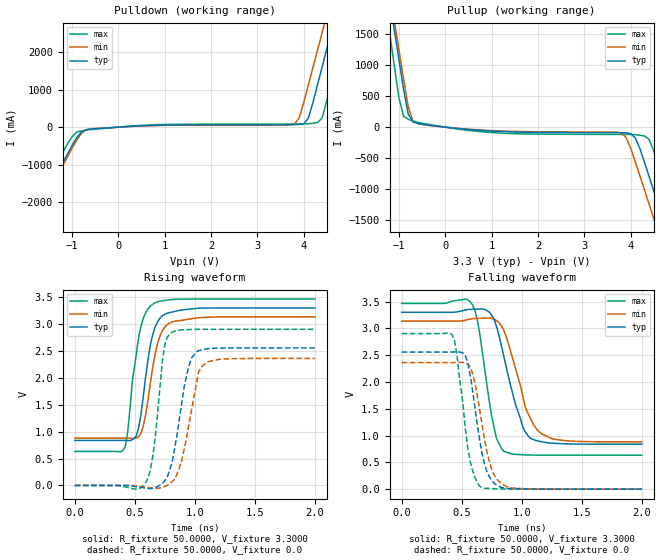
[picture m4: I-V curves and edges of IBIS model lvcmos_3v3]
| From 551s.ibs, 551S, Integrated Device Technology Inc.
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|   Model LVCMOS_3V3
[Model]  lvcmos_3v3
Model_type Output
Polarity   Non-Inverting
Vmeas =  1.6500V
Cref =   5.0000pF
Rref =   50.0000
Vref =   1.6500V
C_comp   2.0000pF   1.5000pF   2.5000pF
[Temperature Range]   55.0000   80.0000   -40.0000
[Voltage Range]   3.3000V   3.1350V   3.4650V
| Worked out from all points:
|   slope of the pulldown table from 0 to 0.495 V, typ, clamps not added: 14.3 ohm
|   slope of the pullup table from 0 to 0.495 V, typ, clamps not added: 13.3 ohm
|   rising waveform, R_fixture 50.0000, V_fixture 3.3000: 20-80 % time 97.8ps typ, 104ps min, 95.8ps max; typ from 0.838 V to 3.3 V
|   rising waveform, R_fixture 50.0000, V_fixture 0.0: 20-80 % time 114ps typ, 121ps min, 78.3ps max; typ from 0 V to 2.56 V
|   falling waveform, R_fixture 50.0000, V_fixture 3.3000: 20-80 % time 170ps typ, 177ps min, 115ps max; typ from 3.3 V to 0.838 V
|   falling waveform, R_fixture 50.0000, V_fixture 0.0: 20-80 % time 109ps typ, 118ps min, 96.2ps max; typ from 2.56 V to 0 V
[Pulldown]
|Voltage   I(typ)   I(min)   I(max)
-3.3V     -5.825A    -5.845A    -5.759A
-2.1V     -3.039A    -3.091A    -2.85A
-1.9V     -2.575A    -2.632A    -2.365A
-900mV    -282.7mA   -349.2mA   -131.5mA
-500mV    -41.4mA    -38.13mA   -55.03mA
3.8V      66.61mA    82.58mA    82.03mA
4.1V      237.1mA    1.123A     90.77mA
4.3V      1.138A     2.061A     122.5mA
4.4V      1.618A     2.53A      248.5mA
4.6V      2.578A     3.468A     1.24A
4.9V      4.02A      4.877A     2.824A
6.6V      12.23A     12.9A      11.85A
[Pullup]
|Voltage   I(typ)   I(min)   I(max)
-3.3V     12.12A     12.03A     12.56A
-1.3V     2.533A     2.657A     2.046A
-1.2V     2.053A     2.188A     1.52A
-1.1V     1.573A     1.719A     994mA
-900mV    613.8mA    780.7mA    174.6mA
-700mV    83.85mA    99.95mA    100.2mA
3.8V      -90.26mA   -92.25mA   -118.4mA
4.1V      -171.8mA   -555.8mA   -121.3mA
4.3V      -566.6mA   -1.015A    -144mA
4.6V      -1.263A    -1.704A    -620mA
5V        -2.193A    -2.624A    -1.593A
6.6V      -5.928A    -6.315A    -5.503A
[Ramp]
| variable   typ   min   max
dV/dt_r  1.5342/0.1142n   1.4166/0.1326n   1.7418/78.2746p
dV/dt_f  1.4771/0.1700n   1.3527/0.1971n   1.6990/0.1147n
R_load = 50.0000
[Rising Waveform]
R_fixture= 50.0000
V_fixture= 3.3000
V_fixture_min= 3.1350
V_fixture_max= 3.4650
|time   V(typ)   V(min)   V(max)
0s        837.6mV    879.8mV    633.2mV
420ps     836.3mV    880.1mV    720.7mV
440ps     833.5mV    879.1mV    982.5mV
480ps     851mV      874.7mV    1.948V
530ps     1.052V     900.9mV    2.731V
590ps     2.011V     1.311V     3.206V
650ps     2.811V     2.212V     3.369V
730ps     3.157V     2.877V     3.432V
830ps     3.232V     3.051V     3.458V
2ns       3.299V     3.134V     3.464V
[Rising Waveform]
R_fixture= 50.0000
V_fixture= 0.0
V_fixture_min= 0.0
V_fixture_max= 0.0
|time   V(typ)   V(min)   V(max)
0s        0V         0V         0V
590ps     -50.04mV   -31.75mV   50.72mV
650ps     -52.51mV   -51.65mV   547.5mV
750ps     90.18mV    -18.72mV   2.615V
810ps     420.2mV    68.05mV    2.848V
930ps     2.031V     870.2mV    2.897V
1.01ns    2.475V     1.854V     2.901V
1.05ns    2.515V     2.191V     2.901V
1.11ns    2.543V     2.3V       2.902V
2ns       2.557V     2.361V     2.903V
[Falling Waveform]
R_fixture= 50.0000
V_fixture= 3.3000
V_fixture_min= 3.1350
V_fixture_max= 3.4650
|time   V(typ)   V(min)   V(max)
0s        3.3V       3.135V     3.465V
590ps     3.355V     3.18V      3.44V
650ps     3.361V     3.187V     2.906V
750ps     3.247V     3.186V     1.362V
790ps     3.04V      3.145V     946.9mV
850ps     2.489V     2.969V     708.7mV
1.01ns    1.159V     1.728V     641.2mV
1.09ns    932.4mV    1.243V     635.9mV
1.17ns    883.2mV    1.027V     634.7mV
2ns       838.1mV    880.5mV    633.4mV
[Falling Waveform]
R_fixture= 50.0000
V_fixture= 0.0
V_fixture_min= 0.0
V_fixture_max= 0.0
|time   V(typ)   V(min)   V(max)
0s        2.557V     2.361V     2.903V
420ps     2.558V     2.361V     2.88V
460ps     2.562V     2.363V     2.522V
550ps     2.364V     2.338V     783.7mV
590ps     1.853V     2.167V     352.3mV
650ps     906.8mV    1.477V     56.24mV
690ps     472.7mV    934.8mV    16.97mV
750ps     166.9mV    375.5mV    10.69mV
850ps     23.64mV    75.35mV    3.857mV
2ns       152.1uV    166.7uV    120uV
